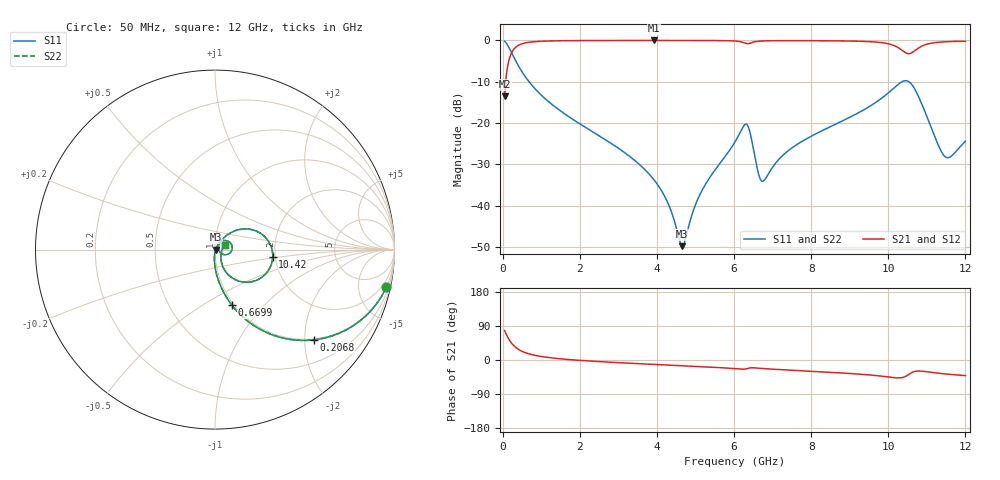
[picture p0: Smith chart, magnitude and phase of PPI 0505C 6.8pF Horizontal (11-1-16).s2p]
# MHz S MA R 50
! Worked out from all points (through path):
!   1601 points, 50 MHz to 12 GHz, reference 50 ohm
!   highest |S21| = -0.03 dB at 3.934 GHz (marker M1); lowest = -13.5 dB at 50 MHz (marker M2)
!   group delay of S21, straight-line fit = 14.5 ps
!   lowest |S11| = -49.8 dB at 4.658 GHz (marker M3), VSWR 1.01, Z = 50.3 - j0.0978 ohm
!   |S11| at or under -10 dB: 683 MHz to 10.36 GHz (9.675 GHz wide, 175 % of centre); 10.53 GHz to end of sweep
!   |S22| runs from -49.8 to -0.2 dB; largest |S21 - S12| = 0
!   S11 on the Smith chart (normalised r, x): 50 MHz: 0.98, -9.15; 206.8 MHz: 0.98, -2.21; 669.9 MHz: 0.98, -0.67; 10.42 GHz: 1.94, -0.19; 12 GHz: 1.11, +0.06
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50  0.9775 -12.3  0.2108 77.7  0.2108 77.7  0.9775 -12.3
206.8438  0.7454 -42.4  0.666 47.5  0.666 47.5  0.7454 -42.4
393.5625  0.5051 -60.9  0.8621 29.0  0.8621 29.0  0.5051 -60.9
669.9062  0.322 -73.2  0.9455 16.6  0.9455 16.6  0.322 -73.2
2044.156  0.09496 -90.1  0.9934 -1.3  0.9934 -1.3  0.09496 -90.1
3933.75  0.02031 -93.9  0.9968 -11.7  0.9968 -11.7  0.02031 -93.9
4038.312  0.01741 -92.9  0.9968 -12.2  0.9968 -12.2  0.01741 -92.9
4322.125  0.009821 -85.9  0.9967 -13.6  0.9967 -13.6  0.009821 -85.9
4658.219  0.003244 -17.4  0.9965 -15.2  0.9965 -15.2  0.003244 -17.4
5151.156  0.01475 57.1  0.9957 -17.6  0.9957 -17.6  0.01475 57.1
6025  0.0592 51.1  0.9816 -22.8  0.9816 -22.8  0.0592 51.1
6346.156  0.09464 -0.4  0.9114 -22.6  0.9114 -22.6  0.09464 -0.4
6637.438  0.02406 -17.4  0.9756 -21.6  0.9756 -21.6  0.02406 -17.4
6749.469  0.01979 13.2  0.9834 -22.5  0.9834 -22.5  0.01979 13.2
7287.219  0.0416 53.7  0.9912 -25.9  0.9912 -25.9  0.0416 53.7
8019.156  0.06994 54.4  0.99 -29.8  0.99 -29.8  0.06994 54.4
10013.31  0.2341 28.3  0.9064 -44.9  0.9064 -44.9  0.2341 28.3
10424.09  0.3245 -7.6  0.7205 -44.4  0.7205 -44.4  0.3245 -7.6
10707.91  0.2468 -47.4  0.7614 -29.7  0.7614 -29.7  0.2468 -47.4
10984.25  0.1256 -64.9  0.8928 -30.8  0.8928 -30.8  0.1256 -64.9
11454.78  0.03995 -29.8  0.9596 -36.5  0.9596 -36.5  0.03995 -29.8
12000  0.06014 27.6  0.9759 -41.1  0.9759 -41.1  0.06014 27.6
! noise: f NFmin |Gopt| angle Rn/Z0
50  0.0005379  0.9054  1.555  0.001247
1372  0.004795  0.7217  4.986  0.003409
2701  0.007845  0.6748  9.122  0.004623
4031  0.01077  0.6528  13.25  0.00583
5360  0.01557  0.6776  17.34  0.009124
6682  0.03651  0.8158  21.62  0.04
8012  0.02375  0.6874  25.51  0.01406
9341  0.04006  0.775  29.62  0.03404
1.067e+04  0.1871  0.9405  33.93  0.6425
1.2e+04  0.05018  0.7745  37.77  0.04077
